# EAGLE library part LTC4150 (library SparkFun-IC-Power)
LTC4150 Coulomb Counter / Battery Gas Gauge Indicates Charge Quantity and Polarity ±50mV Sense Voltage Range Precision Timer Capacitor or Crystal Not Required 2.7V to 8.5V Operation High Side Sense 32.55Hz/V Charge Count Frequency 1.5μA Shutdown Current 10-Pin MSOP Package Datasheet Manufacturer's page: http://www.linear.com/product/LTC4150 SparkFun Products SparkFun Coulomb Counter Breakout - LTC4150 (BOB-12052)
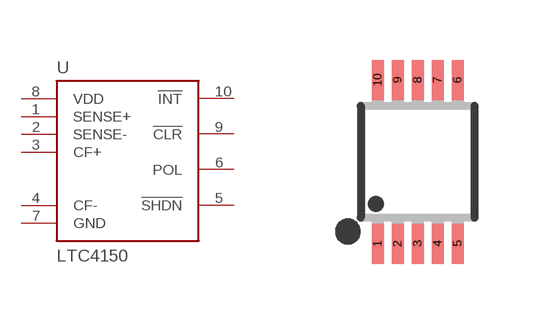
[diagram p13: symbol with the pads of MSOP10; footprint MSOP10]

Designator prefix U

## LTC4150 (PROD_ID: IC-11785; VALUE: LTC4150CMS)  [MSOP10]
1  SENSE+
2  SENSE-
3  CF+
4  CF-
5  !SHDN!  in
6  POL
7  GND  pwr
8  VDD  pwr
9  !CLR!
10  !INT!

## Footprint MSOP10 (pad centres in mm)
10 Lead Platic MSOP Source: http://www.linear.com .. LT1996
smd 0.3 x 1: 1 -1,-2.05; 2 -0.5,-2.05; 3 0,-2.05; 4 0.5,-2.05; 5 1,-2.05; 6 1,2.05; 7 0.5,2.05; 8 0,2.05; 9 -0.5,2.05; 10 -1,2.05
